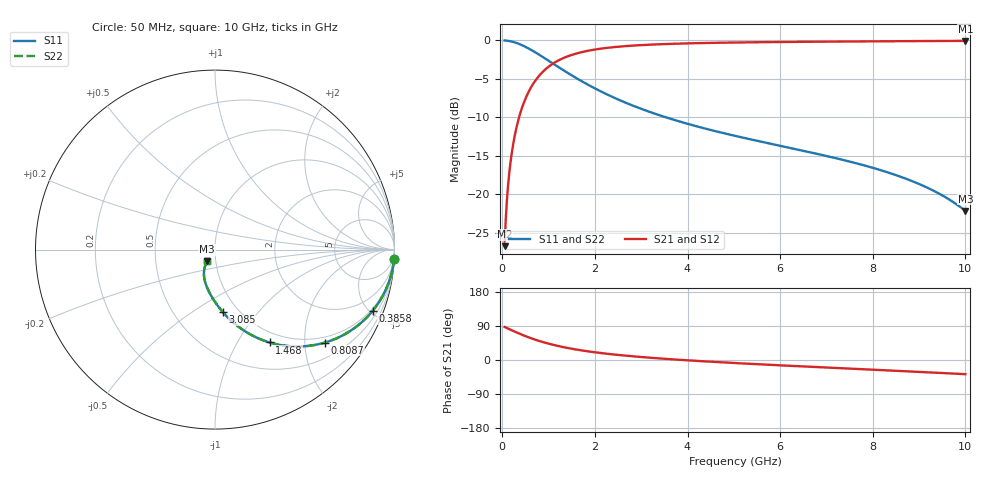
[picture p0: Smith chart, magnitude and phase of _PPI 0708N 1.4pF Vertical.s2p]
! S-Parameter data specifications (vertical orientation):
! Substrate: 40-mil Rogers 3003C, Substrate thickness, H=1.016mm, Dielectric constant, Er=3, Conductor thickness, T_mtl=0.043mm, Loss Tangent, Tand=0.003
! PCB Mounting Pad Footprint: Pad width, PadW=2.54mm , Pad length, PadL=0.51mm , Pad gap, PadG (edge-to-edge)=0.71mm , Reference planes=1.73mm apart
! Created Tue Jan 16 08:43:04 2018
# GHz S MA R 50
! 2 Port Network Data from SP1.SP block
! freq  magS11  angS11  magS21  angS21  magS12  angS12  magS22  angS22
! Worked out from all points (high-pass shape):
!   801 points, 50 MHz to 10 GHz, reference 50 ohm
!   highest |S21| = -0.06 dB at 10 GHz (marker M1); lowest = -26.7 dB at 50 MHz (marker M2)
!   |S21| within 3 dB of the highest: 1.083 GHz to end of sweep
!   lowest |S11| = -22.2 dB at 10 GHz (marker M3), VSWR 1.17, Z = 45.4 - j5.87 ohm
!   |S11| at or under -10 dB: 3.535 GHz to end of sweep
!   |S22| runs from -22.2 to 0.0 dB; largest |S21 - S12| = 0
!   S11 on the Smith chart (normalised r, x): 50 MHz: 1, -40; 385.8 MHz: 0.85, -5.19; 808.7 MHz: 0.85, -2.48; 1.468 GHz: 0.85, -1.38; 3.085 GHz: 0.85, -0.67; 10 GHz: 0.91, -0.12
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0.05  0.9989 -2.9  0.04605 87.1  0.04605 87.1  0.9989 -2.9
0.074875  0.9976 -4.3  0.06887 85.7  0.06887 85.7  0.9976 -4.3
0.1370625  0.9921 -7.8  0.1254 82.2  0.1254 82.2  0.9921 -7.8
0.1868125  0.9855 -10.6  0.1697 79.4  0.1697 79.4  0.9855 -10.6
0.224125  0.9793 -12.7  0.2023 77.3  0.2023 77.3  0.9793 -12.7
0.273875  0.9696 -15.4  0.2447 74.6  0.2447 74.6  0.9696 -15.4
0.3858125  0.9422 -21.3  0.3348 68.7  0.3348 68.7  0.9422 -21.3
0.472875  0.9168 -25.6  0.399 64.4  0.399 64.4  0.9168 -25.6
0.572375  0.8848 -30.3  0.4657 59.7  0.4657 59.7  0.8848 -30.3
0.8086875  0.803 -40.1  0.5955 49.8  0.5955 49.8  0.803 -40.1
1.132062  0.6952 -50.9  0.7182 39.0  0.7182 39.0  0.6952 -50.9
1.467875  0.6004 -59.5  0.7988 30.4  0.7988 30.4  0.6004 -59.5
1.716625  0.5425 -64.6  0.8391 25.3  0.8391 25.3  0.5425 -64.6
2.002687  0.4872 -69.6  0.8722 20.3  0.8722 20.3  0.4872 -69.6
2.313625  0.4382 -74.1  0.8977 15.8  0.8977 15.8  0.4382 -74.1
3.08475  0.3516 -82.8  0.9348 7.0  0.9348 7.0  0.3516 -82.8
3.370812  0.3281 -85.4  0.9432 4.3  0.9432 4.3  0.3281 -85.4
5.025  0.2399 -97.6  0.9689 -8.0  0.9689 -8.0  0.2399 -97.6
6.691625  0.1862 -107.4  0.9801 -18.1  0.9801 -18.1  0.1862 -107.4
8.345812  0.1382 -116.4  0.9873 -27.6  0.9873 -27.6  0.1382 -116.4
9.266187  0.1073 -121.2  0.9906 -32.9  0.9906 -32.9  0.1073 -121.2
10  0.07805 -124.6  0.9928 -37.4  0.9928 -37.4  0.07805 -124.6
